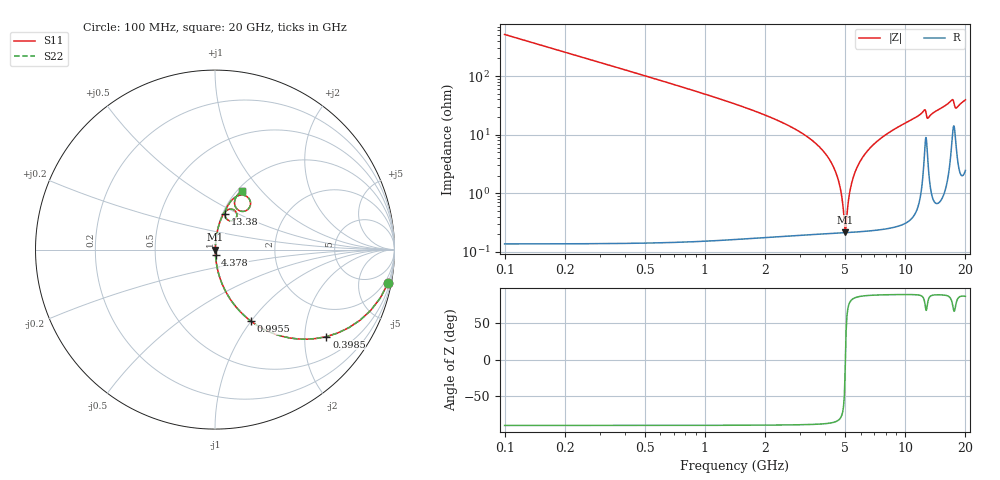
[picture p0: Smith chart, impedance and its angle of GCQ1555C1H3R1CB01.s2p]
!Murata Part Number: GCQ1555C1H3R1CB01
!These Parameters are Measured in Series Mode Connection
!Data Generated on Jan 08, 2026
!  o--ll--o
!Port1  Port2
!  o------o
!Operation Temp=25[degC], DC Bias Voltage=0[V]
!Freq. Start=100[MHz] Stop=20[GHz] 401[Steps]
# Hz S RI R 50
!Freq.(Hz) S11(Real) S11(Imag) S21(Real) S21(Imag) S12(Real) S12(Imag) S22(Real) S22(Imag)
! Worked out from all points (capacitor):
!   401 points, 100 MHz to 20 GHz, reference 50 ohm
!   read as one part in series: C = 3.1 pF near 199.5 MHz
!   lowest |Z| = 215 mohm at 5.025 GHz (marker M1)
!   series resonance near 5.033 GHz, so ESL is about 320 pH
!   S11 on the Smith chart (normalised r, x): 100 MHz: 1, -10; 398.5 MHz: 1.00, -2.56; 995.5 MHz: 1.00, -0.99; 4.378 GHz: 1.00, -0.06; 13.38 GHz: 1.02, +0.43; 20 GHz: 1.05, +0.79
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1e8  0.9634 -0.1877  0.0366 0.1877  0.0366 0.1877  0.9634 -0.1877
3.985e8  0.6209 -0.4846  0.3791 0.4846  0.3791 0.4846  0.6209 -0.4846
6.97e8  0.3432 -0.4738  0.6568 0.4738  0.6568 0.4738  0.3432 -0.4738
9.955e8  0.1978 -0.3968  0.8022 0.3968  0.8022 0.3968  0.1978 -0.3968
1.7915e9  0.0603 -0.2347  0.9397 0.2347  0.9397 0.2347  0.0603 -0.2347
3.43325e9  0.0083 -0.0792  0.9917 0.0792  0.9917 0.0792  0.0083 -0.0792
4.3785e9  0.00288 -0.0284  0.9971 0.0284  0.9971 0.0284  0.00288 -0.0284
4.72675e9  0.00226 -0.0128  0.9977 0.0128  0.9977 0.0128  0.00226 -0.0128
5.02525e9  0.00212 -0.000301  0.9979 0.000301  0.9979 0.000301  0.00212 -0.000301
5.12475e9  0.00215 0.0037  0.9979 -0.0037  0.9979 -0.0037  0.00215 0.0037
5.32375e9  0.00228 0.0115  0.9977 -0.0115  0.9977 -0.0115  0.00228 0.0115
5.62225e9  0.00269 0.0227  0.9973 -0.0227  0.9973 -0.0227  0.00269 0.0227
6.07e9  0.00371 0.0385  0.9963 -0.0385  0.9963 -0.0385  0.00371 0.0385
6.7665e9  0.00609 0.0614  0.9939 -0.0614  0.9939 -0.0614  0.00609 0.0614
1.005e10  0.0275 0.154  0.9725 -0.154  0.9725 -0.154  0.0275 0.154
1.2438e10  0.0914 0.2256  0.9086 -0.2256  0.9086 -0.2256  0.0914 0.2256
1.29355e10  0.0721 0.1644  0.9279 -0.1644  0.9279 -0.1644  0.0721 0.1644
1.338325e10  0.0548 0.2007  0.9452 -0.2007  0.9452 -0.2007  0.0548 0.2007
1.67165e10  0.1361 0.3022  0.8639 -0.3022  0.8639 -0.3022  0.1361 0.3022
1.7413e10  0.1982 0.2531  0.8018 -0.2531  0.8018 -0.2531  0.1982 0.2531
1.79105e10  0.126 0.2229  0.874 -0.2229  0.874 -0.2229  0.126 0.2229
2e10  0.1491 0.3263  0.8509 -0.3263  0.8509 -0.3263  0.1491 0.3263
